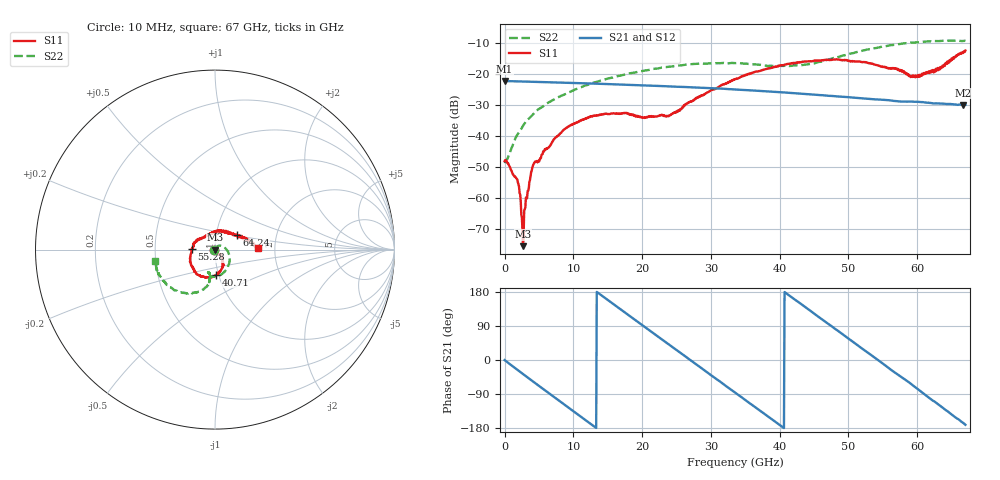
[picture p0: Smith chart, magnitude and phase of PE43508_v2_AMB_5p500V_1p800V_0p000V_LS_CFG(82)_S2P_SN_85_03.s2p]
!Keysight Technologies,N5227A,US51270237,A.10.43.00
!Date: Wednesday, August 22, 2018 17:15:12
!Correction: S11(Full 2 Port(1,3))
!S31(Full 2 Port(1,3))
!S13(Full 2 Port(1,3))
!S33(Full 2 Port(1,3))
!S2P File: Measurements: S11, S31, S13, S33:
# Hz S  dB  R 50
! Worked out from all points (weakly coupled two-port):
!   801 points, 10 MHz to 67 GHz, reference 50 ohm
!   highest |S21| = -22.28 dB at 10 MHz (marker M1); lowest = -30.0 dB at 66.67 GHz (marker M2)
!   lowest |S11| = -75.5 dB at 2.69 GHz (marker M3), VSWR 1.00, Z = 50 + j0.00945 ohm
!   |S11| at or under -10 dB: start of sweep to end of sweep
!   |S22| runs from -48.7 to -9.2 dB; largest |S21 - S12| = 0.0004
!   S11 on the Smith chart (normalised r, x): 10 MHz: 0.99, -0.00; 40.71 GHz: 0.98, -0.28; 55.28 GHz: 0.77, +0.00; 64.24 GHz: 1.25, +0.21; 67 GHz: 1.62, +0.03
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1e7  -48.08 -175.7  -22.28 -0.2  -22.29 -0.2  -48.74 -177.6
1.852225e9  -54.00 153.9  -22.41 -25.7  -22.41 -25.7  -39.60 88.1
2.187175e9  -58.28 161.0  -22.43 -30.3  -22.43 -30.3  -38.53 82.0
2.438388e9  -65.37 163.5  -22.44 -33.7  -22.45 -33.7  -37.69 77.1
2.6896e9  -75.47 34.1  -22.46 -37.1  -22.46 -37.1  -36.76 73.0
2.940812e9  -63.56 11.4  -22.48 -40.5  -22.48 -40.5  -35.90 69.8
3.861925e9  -51.70 -28.1  -22.53 -52.9  -22.54 -52.9  -33.70 59.3
4.36435e9  -48.55 -19.4  -22.56 -59.7  -22.56 -59.7  -32.51 54.7
8.634962e9  -37.96 -60.9  -22.83 -116.9  -22.82 -116.9  -26.70 22.0
1.123082e10  -34.79 -71.4  -23.00 -151.5  -23.01 -151.5  -24.20 3.0
1.583639e10  -32.74 -89.3  -23.35 147.4  -23.35 147.4  -21.07 -24.6
2.236791e10  -33.52 -76.4  -23.89 61.0  -23.89 61.0  -18.20 -56.6
2.395892e10  -33.45 -63.2  -24.03 40.1  -24.03 40.1  -17.67 -63.3
3.3505e10  -21.75 -58.0  -25.02 -86.0  -25.02 -86.0  -16.52 -98.7
4.070642e10  -17.09 -86.6  -25.99 179.3  -25.98 179.3  -17.42 -105.6
4.472582e10  -15.90 -107.1  -26.60 126.3  -26.58 126.4  -16.73 -100.2
5.527675e10  -17.72 179.5  -28.39 -13.2  -28.36 -13.5  -11.13 -119.3
5.586291e10  -18.33 172.5  -28.46 -21.4  -28.45 -21.9  -10.86 -121.5
6.004979e10  -20.43 107.3  -28.96 -76.4  -28.98 -76.7  -9.85 -138.7
6.423666e10  -16.79 33.8  -29.68 -133.2  -29.75 -133.4  -9.28 -157.0
6.666505e10  -13.28 5.8  -29.98 -166.0  -30.05 -166.0  -9.37 -167.6
6.7e10  -12.50 1.8  -29.94 -171.0  -30.02 -170.9  -9.36 -169.4
